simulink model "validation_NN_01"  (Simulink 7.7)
settings: Solver=VariableStepDiscrete  StartTime=0.0  StopTime=100  RelTol=1e-3
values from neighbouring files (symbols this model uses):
  A = [0.9944 -0.1203 -0.4302    [process_model02.m]
  B = [1 0    [process_model02.m]
  C = [1 0 0    [process_model02.m]
  D = zeros(2,2)    [process_model02.m]
  Ts = 0.1    [process_model02.m]
  x0 = [0.01 0.02 0.03]    [process_model02.m]
libraries: neural x21, simulink x6

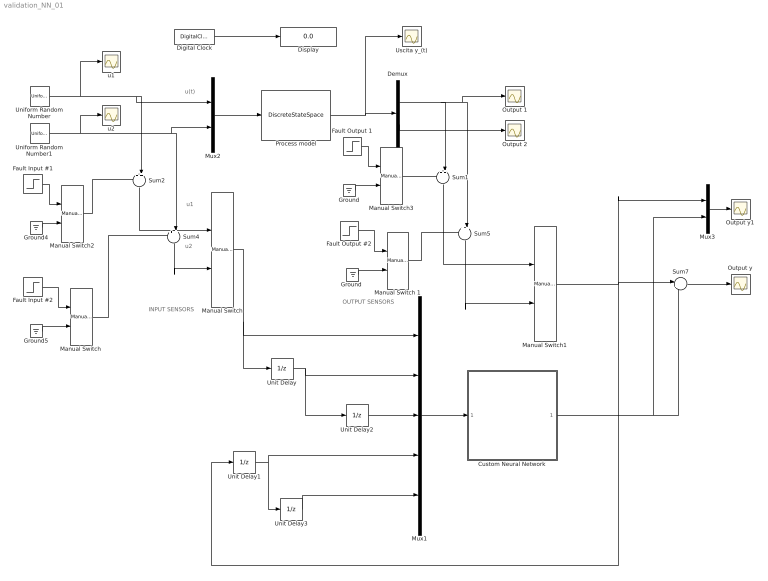
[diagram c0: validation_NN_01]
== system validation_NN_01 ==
  note: u(t)
  note: INPUT SENSORS
  note: OUTPUT SENSORS
  note: u1
  note: u2
  Custom Neural Network : Subsystem
  Demux : Demux  Outputs=2
  Digital Clock : DigitalClock  SampleTime=Ts
  Display : Display
  Fault Input #1 : Step  Time=50  After=5  SampleTime=Ts
  Fault Input #2 : Step  Time=50  After=5  SampleTime=Ts
  Fault Output #2 : Step  Time=50  After=5  SampleTime=Ts
  Fault Output 1 : Step  Time=50  After=100  SampleTime=Ts
  Ground : Ground
  "Ground " : Ground
  Ground4 : Ground
  Ground5 : Ground
  Manual Switch : simulink/Signal Routing/Manual Switch  SystemSampleTime=-1  sw=1  action=0  varsize=off
  "Manual Switch " : simulink/Signal Routing/Manual Switch  SystemSampleTime=-1  sw=0  action=0  varsize=off
  Manual Switch 1 : simulink/Signal Routing/Manual Switch  SystemSampleTime=-1  sw=0  action=0  varsize=off
  Manual Switch1 : simulink/Signal Routing/Manual Switch  SystemSampleTime=-1  sw=1  action=0  varsize=off
  Manual Switch2 : simulink/Signal Routing/Manual Switch  SystemSampleTime=-1  sw=0  action=0  varsize=off
  Manual Switch3 : simulink/Signal Routing/Manual Switch  SystemSampleTime=-1  sw=0  action=0  varsize=off
  Mux1 : Mux  Inputs=5
  Mux2 : Mux  Inputs=2
  Mux3 : Mux  Inputs=2
  Output 1 : Scope
  Output 2 : Scope
  Output y : Scope
  Output y1 : Scope
  Process model : DiscreteStateSpace  A=A  B=B  C=C  D=D  X0=x0  SampleTime=Ts
  Sum{1..2,4..5} (4 alike) : Sum  Inputs=++|
  Sum7 : Sum  Inputs=|+-
  Uniform Random Number : UniformRandomNumber  Seed=11  SampleTime=Ts
  Uniform Random Number1 : UniformRandomNumber  Minimum=-0.5  Maximum=0.5  Seed=13  SampleTime=Ts
  Unit Delay{,1..3} (4 alike) : UnitDelay  SampleTime=Ts
  Uscita y_(t) : Scope
  u1 : Scope
  u2 : Scope
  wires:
  Digital Clock/1 -> Display/1
  Mux2/1 -> Process model/1
  Uniform Random Number/1 -> u1/1, Mux2/1, Sum2/2
  Process model/1 -> Uscita y_(t)/1, Demux/1
  Uniform Random Number1/1 -> u2/1, Mux2/2, Sum4/2
  Demux/1 -> Output 1/1, Sum5/2, Sum1/2
  Demux/2 -> Output 2/1
  Sum2/1 -> Manual Switch/1
  Sum4/1 -> Manual Switch/2
  Manual Switch/1 -> Unit Delay/1, Mux1/1
  Unit Delay/1 -> Unit Delay2/1, Mux1/2
  Sum1/1 -> Manual Switch1/1
  Sum5/1 -> Manual Switch1/2
  Unit Delay1/1 -> Unit Delay3/1, Mux1/4
  Manual Switch1/1 -> Unit Delay1/1, Sum7/1, Mux3/1
  Unit Delay2/1 -> Mux1/3
  Mux1/1 -> Custom Neural Network/1(Input)
  Unit Delay3/1 -> Mux1/5
  Custom Neural Network/1(Output) -> Sum7/2, Mux3/2
  Sum7/1 -> Output y/1
  Mux3/1 -> Output y1/1
  Ground4/1 -> Manual Switch2/2
  Fault Input #1/1 -> Manual Switch2/1
  Fault Input #2/1 -> "Manual Switch "/1
  "Manual Switch "/1 -> Sum4/1
  Manual Switch2/1 -> Sum2/1
  Ground/1 -> Manual Switch3/2
  Fault Output 1/1 -> Manual Switch3/1
  "Ground "/1 -> Manual Switch 1/2
  Fault Output #2/1 -> Manual Switch 1/1
  Manual Switch 1/1 -> Sum5/1
  Manual Switch3/1 -> Sum1/1
  Ground5/1 -> "Manual Switch "/2

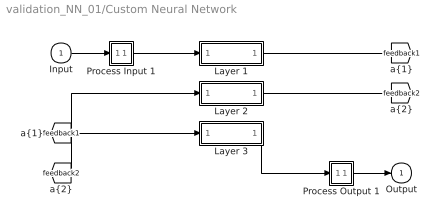
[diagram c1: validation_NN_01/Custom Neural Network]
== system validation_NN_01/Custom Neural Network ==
  Input : Inport  PortDimensions=5
  Layer 1 : Subsystem
  Layer 2 : Subsystem
  Layer 3 : Subsystem
  Process Input 1 : Subsystem
  Process Output 1 : Subsystem
  Output : Outport  InitialOutput=0
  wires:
  Input/1 -> Process Input 1/1(x)
  Process Output 1/1(y) -> Output/1
  Process Input 1/1(p) -> Layer 1/1("p{1}")
  Layer 1/1("a{1}") -> [feedback1]
  [feedback1] -> Layer 2/1("a{1} ")
  Layer 2/1("a{2}") -> [feedback2]
  [feedback2] -> Layer 3/1("a{2} ")
  Layer 3/1("a{3}") -> Process Output 1/1(a)

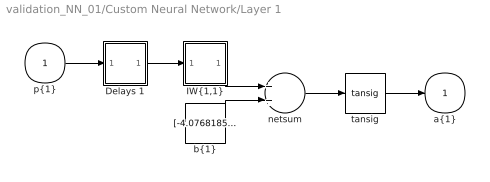
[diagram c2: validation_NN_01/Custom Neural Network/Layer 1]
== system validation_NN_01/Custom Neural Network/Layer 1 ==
  "p{1}" : Inport  PortDimensions=5
  Delays 1 : Subsystem
  "IW{1,1}" : Subsystem
  "b{1}" : Constant  Value=[-4.0768185867947579;-0.98246951013089145;-0.038399821419634834;3.4877363696855594]
  netsum : Sum  Inputs=2
  tansig : neural/Transfer Functions/tansig  SystemSampleTime=-1
  "a{1}" : Outport  InitialOutput=[0;0;0;0]
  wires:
  "p{1}"/1 -> Delays 1/1("p{1}")
  Delays 1/1("pd{1,1}") -> "IW{1,1}"/1("pd{1,1}")
  "IW{1,1}"/1("iz{1,1}") -> netsum/1
  "b{1}"/1 -> netsum/2
  netsum/1 -> tansig/1
  tansig/1 -> "a{1}"/1

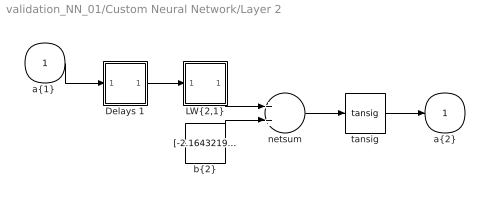
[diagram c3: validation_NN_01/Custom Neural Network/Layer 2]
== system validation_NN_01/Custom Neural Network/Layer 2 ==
  "a{1} " : Inport  PortDimensions=4
  Delays 1 : Subsystem
  "LW{2,1}" : Subsystem
  "b{2}" : Constant  Value=[-2.1643219654493397;-1.3114038341226657;1.7250608115852084;0.73213424846782993;-0.94025775516955057;0.81691600706622569;1.4274902998449444;2.0354503157535877]
  netsum : Sum  Inputs=2
  tansig : neural/Transfer Functions/tansig  SystemSampleTime=-1
  "a{2}" : Outport  InitialOutput=[0;0;0;0;0;0;0;0]
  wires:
  "a{1} "/1 -> Delays 1/1("p{2}")
  Delays 1/1("pd{2,1}") -> "LW{2,1}"/1("ad{2,1}")
  "LW{2,1}"/1("lz{2,1}") -> netsum/1
  "b{2}"/1 -> netsum/2
  netsum/1 -> tansig/1
  tansig/1 -> "a{2}"/1

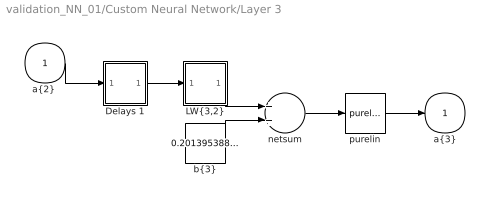
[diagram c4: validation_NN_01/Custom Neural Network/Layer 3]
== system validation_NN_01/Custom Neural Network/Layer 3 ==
  "a{2} " : Inport  PortDimensions=8
  Delays 1 : Subsystem
  "LW{3,2}" : Subsystem
  "b{3}" : Constant  Value=0.20139538814707902
  netsum : Sum  Inputs=2
  purelin : neural/Transfer Functions/purelin  SystemSampleTime=-1
  "a{3}" : Outport  InitialOutput=0
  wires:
  "a{2} "/1 -> Delays 1/1("p{3}")
  Delays 1/1("pd{3,2}") -> "LW{3,2}"/1("ad{3,2}")
  "LW{3,2}"/1("lz{3,2}") -> netsum/1
  "b{3}"/1 -> netsum/2
  netsum/1 -> purelin/1
  purelin/1 -> "a{3}"/1

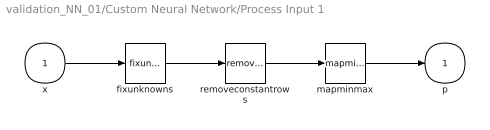
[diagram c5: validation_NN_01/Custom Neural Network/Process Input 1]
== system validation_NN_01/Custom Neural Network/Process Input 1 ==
  x : Inport  PortDimensions=5
  fixunknowns : neural/Processing Functions/fixunknowns  SystemSampleTime=-1  inputSize=5  indices=[1 2 3 4 5]
  mapminmax : neural/Processing Functions/mapminmax  SystemSampleTime=-1  xmin=[-1.137661454327592;-1.1106929140419901;-1.121216738180955;-31.095443858794159;-31.404321949219387]  xmax=[1.1540492640826692;1.122893357889289;1.1111953057620241;32.607744268199028;33.039723432629302]  ymin=-1  ymax=1
  removeconstantrows : neural/Processing Functions/removeconstantrows  SystemSampleTime=-1  inputSize=5  keep=[1 2 3 4 5]
  p : Outport  PortDimensions=5
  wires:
  x/1 -> fixunknowns/1
  fixunknowns/1 -> removeconstantrows/1
  removeconstantrows/1 -> mapminmax/1
  mapminmax/1 -> p/1

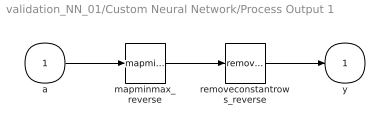
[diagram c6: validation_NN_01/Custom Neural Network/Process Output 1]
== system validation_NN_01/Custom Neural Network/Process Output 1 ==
  a : Inport  PortDimensions=1
  mapminmax_reverse : neural/Processing Functions/mapminmax_reverse  SystemSampleTime=-1  xmin=-31.173256733227603  xmax=32.664397268400201  ymin=-1  ymax=1
  removeconstantrows_reverse : neural/Processing Functions/removeconstantrows_reverse  SystemSampleTime=-1  inputSize=1  constants=zeros(0,1)  rearrange=1
  y : Outport  PortDimensions=1
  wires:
  a/1 -> mapminmax_reverse/1
  mapminmax_reverse/1 -> removeconstantrows_reverse/1
  removeconstantrows_reverse/1 -> y/1

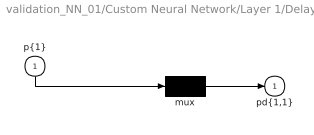
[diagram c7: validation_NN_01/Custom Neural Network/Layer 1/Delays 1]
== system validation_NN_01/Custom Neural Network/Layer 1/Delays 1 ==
  "p{1}" : Inport  PortDimensions=5
  mux : Mux  Inputs=1
  "pd{1,1}" : Outport
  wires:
  "p{1}"/1 -> mux/1
  mux/1 -> "pd{1,1}"/1

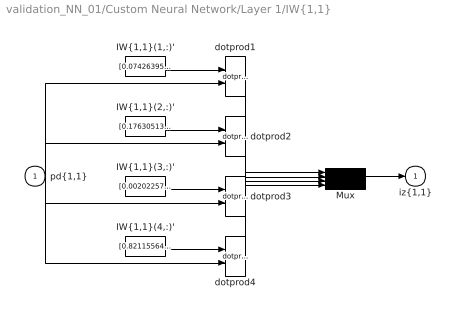
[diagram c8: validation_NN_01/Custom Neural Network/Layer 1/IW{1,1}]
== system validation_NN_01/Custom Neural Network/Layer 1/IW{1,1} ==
  "pd{1,1}" : Inport  PortDimensions=5
  "IW{1,1}(1,:)'" : Constant  Value=[0.074263955351772881;-0.050514147586461534;0.7370437689203122;-0.82946123475770717;1.2551157871936551]
  "IW{1,1}(2,:)'" : Constant  Value=[0.17630513141825749;-0.37512967726353658;-0.62599358893208468;0.34055267402353573;-1.3895246476741532]
  "IW{1,1}(3,:)'" : Constant  Value=[0.0020225785428000633;0.0085945620959656036;-0.0044942734677444716;0.27591694219092405;0.084397730067887061]
  "IW{1,1}(4,:)'" : Constant  Value=[0.82115564213795778;-2.1015791227463634;-1.6313148696872286;0.30992411325126967;0.4625969920876592]
  Mux : Mux
  dotprod{1..4} (4 alike) : neural/Weight Functions/dotprod  SystemSampleTime=-1
  "iz{1,1}" : Outport
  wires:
  "IW{1,1}(1,:)'"/1 -> dotprod1/1
  "pd{1,1}"/1 -> dotprod1/2, dotprod2/2, dotprod3/2, dotprod4/2
  dotprod1/1 -> Mux/1
  "IW{1,1}(2,:)'"/1 -> dotprod2/1
  dotprod2/1 -> Mux/2
  "IW{1,1}(3,:)'"/1 -> dotprod3/1
  dotprod3/1 -> Mux/3
  "IW{1,1}(4,:)'"/1 -> dotprod4/1
  dotprod4/1 -> Mux/4
  Mux/1 -> "iz{1,1}"/1

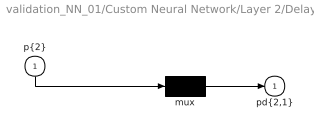
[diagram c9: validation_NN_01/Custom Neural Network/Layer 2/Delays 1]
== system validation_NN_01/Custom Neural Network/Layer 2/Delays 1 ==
  "p{2}" : Inport  PortDimensions=4
  mux : Mux  Inputs=1
  "pd{2,1}" : Outport
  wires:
  "p{2}"/1 -> mux/1
  mux/1 -> "pd{2,1}"/1

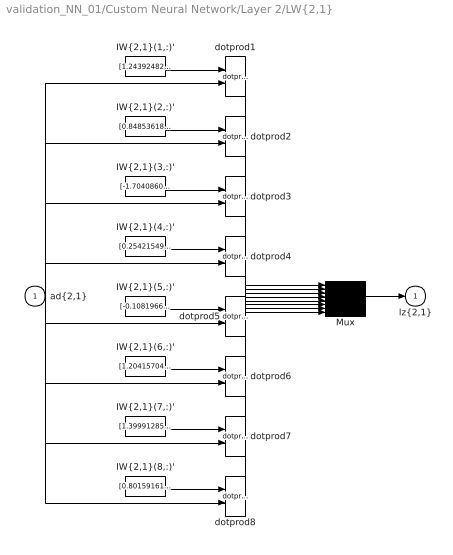
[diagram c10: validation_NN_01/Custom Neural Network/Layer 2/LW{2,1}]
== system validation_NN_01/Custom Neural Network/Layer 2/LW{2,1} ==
  "ad{2,1}" : Inport  PortDimensions=4
  "IW{2,1}(1,:)'" : Constant  Value=[1.2439248254679363;-1.5675910018278842;1.3354404193062686;0.14350495580986344]
  "IW{2,1}(2,:)'" : Constant  Value=[0.84853618115516816;0.82051641032751566;-1.470101414657895;-1.5657936244108774]
  "IW{2,1}(3,:)'" : Constant  Value=[-1.7040860968749072;1.4489672111274152;1.8160180772105508;-1.3222992798410147]
  "IW{2,1}(4,:)'" : Constant  Value=[0.25421549416598899;-1.4353628940238203;-1.5327369258164119;-1.5868369579379678]
  "IW{2,1}(5,:)'" : Constant  Value=[-0.10819667240933188;-1.062287402911223;0.19978015879168601;1.0183121674891378]
  "IW{2,1}(6,:)'" : Constant  Value=[1.2041570478748698;0.19376343529351986;1.9782283626149562;-0.1976006332424721]
  "IW{2,1}(7,:)'" : Constant  Value=[1.399912853371204;1.8082955770438229;1.0478763388115599;0.26360136489237918]
  "IW{2,1}(8,:)'" : Constant  Value=[0.80159161198880158;0.25383058402707936;1.9771817784867725;-0.2652869095531375]
  Mux : Mux  Inputs=8
  dotprod{1..8} (8 alike) : neural/Weight Functions/dotprod  SystemSampleTime=-1
  "lz{2,1}" : Outport
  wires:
  "IW{2,1}(1,:)'"/1 -> dotprod1/1
  "ad{2,1}"/1 -> dotprod1/2, dotprod2/2, dotprod3/2, dotprod4/2, dotprod5/2, dotprod6/2, dotprod7/2, dotprod8/2
  dotprod1/1 -> Mux/1
  "IW{2,1}(2,:)'"/1 -> dotprod2/1
  dotprod2/1 -> Mux/2
  "IW{2,1}(3,:)'"/1 -> dotprod3/1
  dotprod3/1 -> Mux/3
  "IW{2,1}(4,:)'"/1 -> dotprod4/1
  dotprod4/1 -> Mux/4
  "IW{2,1}(5,:)'"/1 -> dotprod5/1
  dotprod5/1 -> Mux/5
  "IW{2,1}(6,:)'"/1 -> dotprod6/1
  dotprod6/1 -> Mux/6
  "IW{2,1}(7,:)'"/1 -> dotprod7/1
  dotprod7/1 -> Mux/7
  "IW{2,1}(8,:)'"/1 -> dotprod8/1
  dotprod8/1 -> Mux/8
  Mux/1 -> "lz{2,1}"/1

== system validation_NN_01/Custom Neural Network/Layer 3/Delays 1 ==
  "p{3}" : Inport  PortDimensions=8
  mux : Mux  Inputs=1
  "pd{3,2}" : Outport
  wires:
  "p{3}"/1 -> mux/1
  mux/1 -> "pd{3,2}"/1

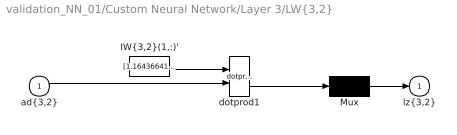
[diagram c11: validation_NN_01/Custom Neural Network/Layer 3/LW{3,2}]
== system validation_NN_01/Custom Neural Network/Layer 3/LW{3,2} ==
  "ad{3,2}" : Inport  PortDimensions=8
  "IW{3,2}(1,:)'" : Constant  Value=[1.1643664181660411;-0.78162354431733683;-0.26793196275406361;-0.017869435906933351;0.2842816660312022;1.0213999315624551;-0.024857354400431617;1.3128539953145097]
  Mux : Mux  Inputs=1
  dotprod1 : neural/Weight Functions/dotprod  SystemSampleTime=-1
  "lz{3,2}" : Outport
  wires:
  "IW{3,2}(1,:)'"/1 -> dotprod1/1
  "ad{3,2}"/1 -> dotprod1/2
  dotprod1/1 -> Mux/1
  Mux/1 -> "lz{3,2}"/1
